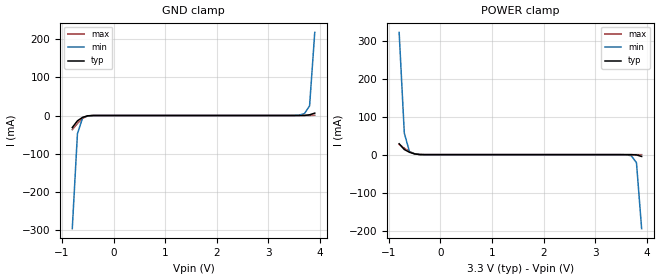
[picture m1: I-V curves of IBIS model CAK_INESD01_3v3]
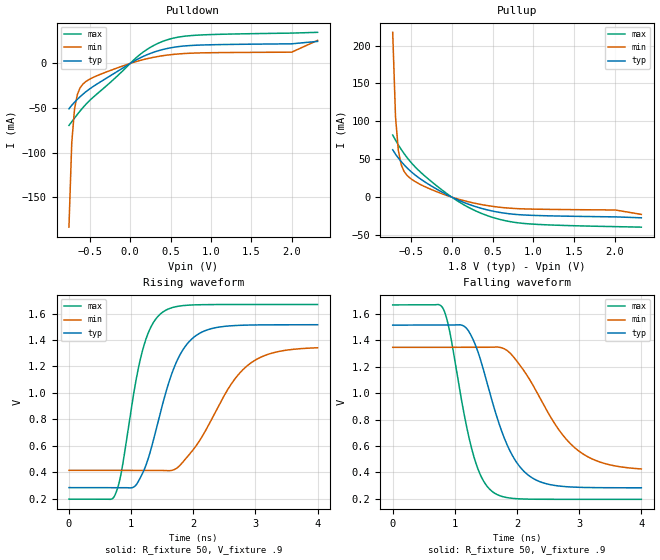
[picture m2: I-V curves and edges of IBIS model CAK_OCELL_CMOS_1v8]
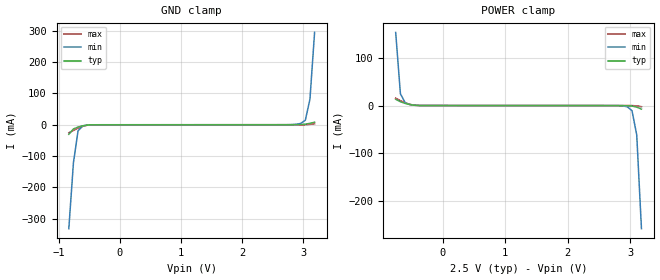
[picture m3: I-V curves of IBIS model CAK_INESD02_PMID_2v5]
|   This file is an IBIS representation of the   |
|   Integrated Device Technology Inc   |
|   IDT8T49N285I   |
|   FEMTOCLOCK NG OCTAL UNIVERSAL FREQUENCY TRANSLATOR   |
[IBIS Ver]   4.1
[File name]   8t49n285i.ibs
[File Rev]   1.0
[Date]   04 Dec 2014
[Source]   Originated at Integrated Device Technology, Inc.
[Disclaimer]
IDT hereby grants the user of this IBIS model a non-exclusive,
nontransferable license to use this IBIS model under the following terms.
Before using this IBIS model, the user should read this license.
If the user does not accept these terms,  the IBIS model should be
returned to IDT within 30 days.
   The user is granted this license only to use the IBIS model and
is not granted rights to sell, load, rent, lease or license the IBIS
model in whole or in part, or in modified form to anyone other than
user. User may modify the IBIS model to suit its specific
applications but rights to derivative works and such modifications
shall belong to IDT.
   This IBIS model is provided on an "AS IS" basis and IDT makes
absolutely no warranty with respect to the information contained
herein. IDT DISCLAIMS AND CUSTOMER WAIVES ALL WARRANTIES, EXPRESS
OR IMPLIED, INCLUDING WARRANTIES OF MERCHANTABILITY OR FITNESS FOR
A PARTICULAR PURPOSE. The entire risk as to quality and performance
is with the Customer. ACCORDINGLY, IN NO EVENT SHALL THE COMPANY BE
LIABLE FOR ANY DAMAGES, WHETHER IN CONTRACT OR TORT,INCLUDING ANY
LOST PROFITS OR OTHER INCIDENTAL, CONSEQUENTIAL, EXEMPLARY, OR
PUNITIVE DAMAGES ARISING OUT OF THE USE OR APPLICATION OF THE IBIS
model provided in this package. Further, IDT reserves the right to
make changes without notice to any product herein to improve
reliability, function, or design. IDT does not convey any license
under patent rights or any other intellectual property rights,
including those of third parties.
   IDT is not obligated to provide maintenance or support
for the licensed IBIS model.
[Copyright] Copyright 2014 by Integrated Device Technology, Inc.
[Component]   IDT8T49N285NLI
[Manufacturer] Integrated Device Technology, Inc.
[Package]
|LD QFN 56
|lead + wire   typ   min   max
R_pkg   294.15m   250.8m   337.5m
L_pkg   1.827nH   1.475nH   2.179nH
C_pkg   0.464pF   0.409pF   0.518pF
[Pin] signal_name model_name   R_pin   L_pin   C_pin
1  VCCA   POWER   337.50m   2.179n   0.518p
2  VCCA   POWER   323.05m   2.062n   0.500p
3  OSCI   CAK_INESD01   308.60m   1.944n   0.482p
4  OSCO   NC   294.15m   1.827n   0.464p
5  S_A0   CAK_INESD02_PD   279.70m   1.709n   0.446p
6  VEE   GND   265.25m   1.592n   0.427p
7  CLK0   CAK_INESD02_PD   250.80m   1.475n   0.409p
8  nCLKO   CAK_INESD02_PMID   250.80m   1.475n   0.409p
9  CLK1   CAK_INESD02_PD   265.25m   1.592n   0.427p
10 nCLK1   CAK_INESD02_PMID   279.70m   1.709n   0.446p
11 VCC   POWER   294.15m   1.827n   0.464p
12 SDATA   CAK_IOCMOS35OHM0   308.60m   1.944n   0.482p
13 SCLK   CAK_IOCMOS35OHM0   323.05m   2.062n   0.500p
14 VCCA   POWER   337.50m   2.179n   0.518p
15 VCCA   POWER   337.50m   2.179n   0.518p
16 VCCA   POWER   323.05m   2.062n   0.500p
17 VCC   POWER   308.60m   1.944n   0.482p
18 CAP1   NC   294.15m   1.827n   0.464p
19 CAP1_REF   NC   279.70m   1.709n   0.446p
20 VCCA   POWER   265.25m   1.592n   0.427p
21 GPI01   CAK_IOCMOS25OHM0   250.80m   1.475n   0.409p
22 VCCO3   POWER   250.80m   1.475n   0.409p
23 Q3   CAK_OCELL_MULTOUT   265.25m   1.592n   0.427p
24 nQ3   CAK_OCELL_MULTOUT   279.70m   1.709n   0.446p
25 GPIO0   CAK_IOCMOS25OHM0   294.15m   1.827n   0.464p
26 VCCO2   POWER   308.60m   1.944n   0.482p
27 Q2   CAK_OCELL_MULTOUT   323.05m   2.062n   0.500p
28 nQ2   CAK_OCELL_MULTOUT   337.50m   2.179n   0.518p
29 GPIO3   CAK_IOCMOS25OHM0   337.50m   2.179n   0.518p
30 nQ7   CAK_OCELL_MULTOUT   323.05m   2.062n   0.500p
31 Q7   CAK_OCELL_MULTOUT   308.60m   1.944n   0.482p
32 VCCO7   POWER   294.15m   1.827n   0.464p
33 nQ6   CAK_OCELL_MULTOUT   279.70m   1.709n   0.446p
34 Q6   CAK_OCELL_MULTOUT   265.25m   1.592n   0.427p
35 VCCO6   POWER   250.80m   1.475n   0.409p
36 nQ5   CAK_OCELL_MULTOUT   250.80m   1.475n   0.409p
37 Q5   CAK_OCELL_MULTOUT   265.25m   1.592n   0.427p
38 VCCO5   POWER   279.70m   1.709n   0.446p
39 nQ4   CAK_OCELL_MULTOUT   294.15m   1.827n   0.464p
40 Q4   CAK_OCELL_MULTOUT   308.60m   1.944n   0.482p
41 VCCO4   POWER   323.05m   2.062n   0.500p
42 GPIO2   CAK_IOCMOS25OHM0   337.50m   2.179n   0.518p
43 nQ1   CAK_OCELL_MULTOUT   337.50m   2.179n   0.518p
44 Q1   CAK_OCELL_MULTOUT   323.05m   2.062n   0.500p
45 VCCO1   POWER   308.60m   1.944n   0.482p
46 nRST   CAK_INESD01_PU_5   294.15m   1.827n   0.464p
47 nQ0   CAK_OCELL_MULTOUT   279.70m   1.709n   0.446p
48 Q0   CAK_OCELL_MULTOUT   265.25m   1.592n   0.427p
49 VCCO0   POWER   250.80m   1.475n   0.409p
50 nINT   OUTPUT_OD01   250.80m   1.475n   0.409p
51 VCCA   POWER   265.25m   1.592n   0.427p
52 CAP0_REF   NC   279.70m   1.709n   0.446p
53 CAP0   NC   294.15m   1.827n   0.464p
54 PLL_BYP   CAK_INESD01_PD_5   308.60m   1.944n   0.482p
55 VCCA   POWER   323.05m   2.062n   0.500p
56 VCCA   POWER   337.50m   2.179n   0.518p
[Diff Pin]   inv_pin vdiff   tdelay_typ   tdelay_min   tdelay_max
| Inputs
7   8   150mV   NA   NA   NA
9   10   150mV   NA   NA   NA
|Outputs
23   24   NA   0   0   0
27   28   NA   0   0   0
31   30   NA   0   0   0
34   33   NA   0   0   0
37   36   NA   0   0   0
40   39   NA   0   0   0
44   43   NA   0   0   0
48   47   NA   0   0   0
[Model Selector] CAK_INESD01
CAK_INESD01_2v5   Buffer selection for 2v5
CAK_INESD01_3v3   Buffer selection for 3v3
[Model Selector] CAK_INESD02_PD
CAK_INESD02_PD_2v5  Buffer selection for 2v5
CAK_INESD02_PD_3v3  Buffer selection for 3v3
[Model Selector] CAK_INESD02_PMID
CAK_INESD02_PMID_2v5  Buffer selection for 2v5
CAK_INESD02_PMID_3v3  Buffer selection for 3v3
[Model Selector] CAK_IOCMOS35OHM0
CAK_IOCMOS35OHM0_2v5  Buffer selection for 2v5
CAK_IOCMOS35OHM0_3v3  Buffer selection for 3v3
[Model Selector] CAK_IOCMOS25OHM0
CAK_IOCMOS25OHM0_2v5  Buffer selection for 2v5
CAK_IOCMOS25OHM0_3v3  Buffer selection for 3v3
[Model Selector] CAK_OCELL_MULTOUT
CAK_OCELL_LVPECL_2v5  Buffer selection for LVPECL 2.5V
CAK_OCELL_LVPECL_3v3  Buffer selection for LVPECL 3.3V
CAK_OCELL_LVDS_2v5   Buffer selection for LVDS 2.5V
CAK_OCELL_LVDS_3v3   Buffer selection for LVDS 3.3V
CAK_OCELL_CMOS_1v8   Buffer selection for CMOS 1.8V
CAK_OCELL_CMOS_2v5   Buffer selection for CMOS 2.5V
CAK_OCELL_CMOS_3v3   Buffer selection for CMOS 3.3V
CAK_OCELL_HCSL_2v5   Buffer selection for HCSL 2.5V
CAK_OCELL_HCSL_3v3   Buffer selection for HCSL 3.3V
[Model Selector] CAK_INESD01_PU_5
CAK_INESD01_PU_5_2v5  Buffer selection for 2v5
CAK_INESD01_PU_5_3v3  Buffer selection for 3v3
[Model Selector] OUTPUT_OD01
OUTPUT_OD01_2v5  Buffer selection for 2v5
OUTPUT_OD01_3v3  Buffer selection for 3v3
[Model Selector] CAK_INESD01_PD_5
CAK_INESD01_PD_5_2v5  Buffer selection for 2v5
CAK_INESD01_PD_5_3v3  Buffer selection for 3v3
| Models and submodels in the file (25): CAK_INESD01_3v3 (Input), CAK_INESD01_2v5 (Input), CAK_OCELL_CMOS_1v8 (Output), CAK_INESD02_PD_2v5 (Input), CAK_INESD02_PMID_2v5 (Input), CAK_IOCMOS35OHM0_2v5 (I/O), CAK_IOCMOS25OHM0_2v5 (I/O), CAK_OCELL_LVPECL_2v5 (Output_ECL), CAK_OCELL_CMOS_2v5 (Output), CAK_OCELL_LVDS_2v5 (Output), CAK_INESD01_PU_5_2v5 (Input), OUTPUT_OD01_2v5 (Open_drain), CAK_INESD01_PD_5_2v5 (Input), CAK_INESD02_PD_3v3 (Input), CAK_INESD02_PMID_3v3 (Input), CAK_IOCMOS35OHM0_3v3 (Output), CAK_IOCMOS25OHM0_3v3 (I/O), CAK_OCELL_LVPECL_3v3 (Output_ECL), CAK_OCELL_CMOS_3v3 (Output), CAK_OCELL_LVDS_3v3 (Output), CAK_INESD01_PU_5_3v3 (Input), OUTPUT_OD01_3v3 (Open_drain), CAK_INESD01_PD_5_3v3 (Input), CAK_OCELL_HCSL_3v3 (Open_source), CAK_OCELL_HCSL_2v5 (Open_source)
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[Model]   CAK_INESD01_3v3
Model_type   Input
Polarity   Non-Inverting
Vinl = 0.8V
Vinh = 2.0V
|   typ   min   max
C_comp   2pF   1.5pF   2.5pF
|   typ   min   max
[Voltage range]   3.3V   3.135V   3.465V
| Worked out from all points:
|   GND clamp passes 1 mA (typ) near -0.51 V on its own axis
|   POWER clamp passes 1 mA (typ) near -0.45 V on its own axis
[GND_clamp]
|Voltage   I (typ)   I (min)   I (max)
|Note, modeling breaks down at 250mA and above.  This is well beyond the functional   |
|operating range of the device.  Should this scenario occur, catastrophic failure and   |
|possible damage to the device and/or board is of higher concern than the I-V curve   |
|behavior.  The IBIS checker will flag currents in excess of 10A with warnings.  Lines   |
|with currents in excess of 0.35 A have been commented out.  The points still remain|
|available to the user if the user desires to use them.   |
|-3.30000e+00   -9.36876e+00   -7.41789e+00   -1.15553e+01
|-3.20000e+00   -8.98667e+00   -7.13115e+00   -1.10681e+01
|-3.10000e+00   -8.60459e+00   -6.84449e+00   -1.05809e+01
|-3.00000e+00   -8.22253e+00   -6.55791e+00   -1.00936e+01
|-2.90000e+00   -7.84049e+00   -6.27142e+00   -9.60637e+00
|-2.80000e+00   -7.45848e+00   -5.98504e+00   -9.11911e+00
|-2.70000e+00   -7.07651e+00   -5.69875e+00   -8.63183e+00
|-2.60000e+00   -6.69459e+00   -5.41259e+00   -8.14455e+00
|-2.50000e+00   -6.31272e+00   -5.12654e+00   -7.65728e+00
|-2.40000e+00   -5.93093e+00   -4.84063e+00   -7.17002e+00
|-2.30000e+00   -5.54921e+00   -4.55486e+00   -6.68278e+00
|-2.20000e+00   -5.16760e+00   -4.26925e+00   -6.19558e+00
|-2.10000e+00   -4.78610e+00   -3.98381e+00   -5.70844e+00
|-2.00000e+00   -4.40474e+00   -3.69855e+00   -5.22138e+00
|-1.90000e+00   -4.02353e+00   -3.41349e+00   -4.73442e+00
|-1.80000e+00   -3.64251e+00   -3.12864e+00   -4.24759e+00
|-1.70000e+00   -3.26171e+00   -2.84402e+00   -3.76091e+00
|-1.60000e+00   -2.88116e+00   -2.55965e+00   -3.27441e+00
|-1.50000e+00   -2.50090e+00   -2.27553e+00   -2.78813e+00
|-1.40000e+00   -2.12097e+00   -1.99169e+00   -2.30210e+00
|-1.30000e+00   -1.74142e+00   -1.70814e+00   -1.81640e+00
|-1.20000e+00   -1.36229e+00   -1.42490e+00   -1.33109e+00
|-1.10000e+00   -9.83643e-01   -1.14199e+00   -8.46264e-01
|-1.00000e+00   -6.05524e-01   -8.59476e-01   -3.62007e-01
|-9.00000e-01   -2.28002e-01   -5.77494e-01   -5.70861e-02
-800mV    -31.5mA    -296.3mA   -37.03mA
-700mV    -13.94mA   -47.89mA   -20.77mA
-600mV    -4.814mA   -5.925mA   -7.477mA
-500mV    -769.5uA   -876.2uA   -1.11mA
-400mV    -50.39uA   -91.12uA   -52.98uA
3.4V      929.4pA    7.738uA    18.23pA
3.6V      7.536uA    1.177mA    576.1pA
3.7V      200.6uA    4.949mA    206.1nA
3.8V      1.845mA    25.21mA    18.18uA
3.9V      6.193mA    217.6mA    563.4uA
| 4.00000e+00   1.34293e-02   5.06540e-01   3.84286e-03
| 4.10000e+00   2.85679e-02   7.94900e-01   1.06020e-02
| 4.20000e+00   2.42102e-01   1.08355e+00   2.05441e-02
| 4.30000e+00   6.27135e-01   1.37257e+00   3.02103e-02
| 4.40000e+00   1.01263e+00   1.66196e+00   7.70913e-02
| 4.50000e+00   1.39863e+00   1.95172e+00   5.37431e-01
| 4.60000e+00   1.78513e+00   2.24185e+00   1.03062e+00
| 4.70000e+00   2.17212e+00   2.53235e+00   1.52443e+00
| 4.80000e+00   2.55958e+00   2.82322e+00   2.01885e+00
| 4.90000e+00   2.94751e+00   3.11446e+00   2.51386e+00
| 5.00000e+00   3.33588e+00   3.40606e+00   3.00943e+00
| 5.10000e+00   3.72470e+00   3.69803e+00   3.50553e+00
| 5.20000e+00   4.11396e+00   3.99038e+00   4.00216e+00
| 5.30000e+00   4.50363e+00   4.28310e+00   4.49928e+00
| 5.40000e+00   4.89373e+00   4.57620e+00   4.99688e+00
| 5.50000e+00   5.28425e+00   4.86969e+00   5.49495e+00
| 5.60000e+00   5.67518e+00   5.16358e+00   5.99346e+00
| 5.70000e+00   6.06653e+00   5.45787e+00   6.49241e+00
| 5.80000e+00   6.45829e+00   5.75259e+00   6.99179e+00
| 5.90000e+00   6.85048e+00   6.04774e+00   7.49160e+00
| 6.00000e+00   7.24309e+00   6.34335e+00   7.99183e+00
| 6.10000e+00   7.63615e+00   6.63943e+00   8.49248e+00
| 6.20000e+00   8.02966e+00   6.93599e+00   8.99355e+00
| 6.30000e+00   8.42363e+00   7.23307e+00   9.49506e+00
| 6.40000e+00   8.81808e+00   7.53069e+00   9.99700e+00
| 6.50000e+00   9.21303e+00   7.82887e+00   1.04994e+01
| 6.60000e+00   9.60850e+00   8.12763e+00   1.10022e+01
[Power_clamp]
|Voltage   I (typ)   I (min)   I (max)
|Note, modeling breaks down at 250mA and above.  This is well beyond the functional   |
|operating range of the device.  Should this scenario occur, catastrophic failure and   |
|possible damage to the device and/or board is of higher concern than the I-V curve   |
|behavior.  The IBIS checker will flag currents in excess of 10A with warnings.  Lines   |
|with currents in excess of 0.35 A have been commented out.  The points still remain|
|available to the user if the user desires to use them.   |
|-3.30000e+00   9.60850e+00   7.63797e+00   1.18330e+01
|-3.20000e+00   9.21303e+00   7.34015e+00   1.13293e+01
|-3.10000e+00   8.81808e+00   7.04288e+00   1.08262e+01
|-3.00000e+00   8.42363e+00   6.74613e+00   1.03235e+01
|-2.90000e+00   8.02966e+00   6.44988e+00   9.82127e+00
|-2.80000e+00   7.63615e+00   6.15411e+00   9.31948e+00
|-2.70000e+00   7.24309e+00   5.85879e+00   8.81813e+00
|-2.60000e+00   6.85048e+00   5.56392e+00   8.31720e+00
|-2.50000e+00   6.45829e+00   5.26948e+00   7.81670e+00
|-2.40000e+00   6.06653e+00   4.97544e+00   7.31662e+00
|-2.30000e+00   5.67518e+00   4.68181e+00   6.81696e+00
|-2.20000e+00   5.28425e+00   4.38857e+00   6.31773e+00
|-2.10000e+00   4.89373e+00   4.09571e+00   5.81893e+00
|-2.00000e+00   4.50363e+00   3.80323e+00   5.32057e+00
|-1.90000e+00   4.11396e+00   3.51113e+00   4.82267e+00
|-1.80000e+00   3.72470e+00   3.21939e+00   4.32523e+00
|-1.70000e+00   3.33588e+00   2.92802e+00   3.82828e+00
|-1.60000e+00   2.94751e+00   2.63702e+00   3.33184e+00
|-1.50000e+00   2.55958e+00   2.34639e+00   2.83591e+00
|-1.40000e+00   2.17212e+00   2.05612e+00   2.34054e+00
|-1.30000e+00   1.78513e+00   1.76623e+00   1.84573e+00
|-1.20000e+00   1.39863e+00   1.47670e+00   1.35152e+00
|-1.10000e+00   1.01263e+00   1.18756e+00   8.57930e-01
|-1.00000e+00   6.27135e-01   8.98775e-01   3.64964e-01
|-9.00000e-01   2.42102e-01   6.10330e-01   4.20775e-02
-800mV    28.57mA    321.9mA    27.12mA
-700mV    13.43mA    56.36mA    16.78mA
-600mV    6.193mA    8.187mA    7.847mA
-500mV    1.845mA    2.071mA    2.293mA
-300mV    7.536uA    23.16uA    4.595uA
3.5V      -38.15nA   -37.11uA   -1.389nA
3.7V      -50.39uA   -3.041mA   -40.99nA
3.8V      -769.5uA   -21.19mA   -4.022uA
3.9V      -4.814mA   -194.9mA   -172.8uA
| 3.25758e+00   -2.17526e-02   -5.28437e-01   -1.11612e-02
| 3.33333e+00   -5.02557e-02   -7.41905e-01   -2.20995e-02
| 3.40909e+00   -2.62296e-01   -9.55738e-01   -3.45860e-02
| 3.48485e+00   -5.48283e-01   -1.16984e+00   -4.61839e-02
| 3.56061e+00   -8.34620e-01   -1.38416e+00   -9.03549e-02
| 3.63636e+00   -1.12128e+00   -1.59867e+00   -4.17005e-01
| 3.71212e+00   -1.40822e+00   -1.81336e+00   -7.83863e-01
| 3.78788e+00   -1.69544e+00   -2.02823e+00   -1.15106e+00
| 3.86364e+00   -1.98290e+00   -2.24326e+00   -1.51854e+00
| 3.93939e+00   -2.27059e+00   -2.45845e+00   -1.88629e+00
| 4.01515e+00   -2.55849e+00   -2.67380e+00   -2.25425e+00
| 4.09091e+00   -2.84658e+00   -2.88929e+00   -2.62240e+00
| 4.16667e+00   -3.13483e+00   -3.10491e+00   -2.99072e+00
| 4.24242e+00   -3.42324e+00   -3.32067e+00   -3.35917e+00
| 4.31818e+00   -3.71177e+00   -3.53656e+00   -3.72774e+00
| 4.39394e+00   -4.00043e+00   -3.75256e+00   -4.09641e+00
| 4.46970e+00   -4.28920e+00   -3.96868e+00   -4.46517e+00
| 4.54545e+00   -4.57807e+00   -4.18490e+00   -4.83401e+00
| 4.62121e+00   -4.86701e+00   -4.40122e+00   -5.20293e+00
| 4.69697e+00   -5.15604e+00   -4.61763e+00   -5.57191e+00
| 4.77273e+00   -5.44513e+00   -4.83413e+00   -5.94093e+00
| 4.84848e+00   -5.73428e+00   -5.05072e+00   -6.31000e+00
| 4.92424e+00   -6.02348e+00   -5.26738e+00   -6.67909e+00
| 5.00000e+00   -6.31272e+00   -5.48412e+00   -7.04821e+00
[Model]   CAK_OCELL_CMOS_1v8
Model_type   Output
Polarity   Non-Inverting
|   typ   min   max
C_comp   2pF   1.5pF   2.5pF
Vmeas = .9
Rref = 50
Cref = 0
Vref = .9
|   typ   min   max
[Voltage range]   1.8V   1.710V   1.890V
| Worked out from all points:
|   slope of the pulldown table from 0 to 0.27 V, typ, clamps not added: 22.7 ohm
|   slope of the pullup table from 0 to 0.27 V, typ, clamps not added: 22.9 ohm
|   rising waveform, R_fixture 50, V_fixture .9: 20-80 % time 472ps typ, 713ps min, 340ps max; typ from 0.284 V to 1.51 V
|   falling waveform, R_fixture 50, V_fixture .9: 20-80 % time 521ps typ, 753ps min, 370ps max; typ from 1.51 V to 0.284 V
[Pulldown]
|Voltage   I (typ)   I (min)   I (max)
|Note, modeling breaks down at 250mA and above.  This is well beyond the functional   |
|operating range of the device.  Should this scenario occur, catastrophic failure and   |
|possible damage to the device and/or board is of higher concern than the I-V curve   |
|behavior.  The IBIS checker will flag currents in excess of 10A with warnings.  Lines   |
|with currents in excess of 0.35 A have been commented out.  The points still remain|
|available to the user if the user desires to use them.   |
|-1.64000e+00   -8.45060e+00   -7.45572e+00   -9.66339e+00
|-1.48000e+00   -6.67178e+00   -6.12326e+00   -7.39014e+00
|-1.32000e+00   -4.89321e+00   -4.79099e+00   -5.11762e+00
|-1.16000e+00   -3.11502e+00   -3.45890e+00   -2.84539e+00
|-1.00000e+00   -1.33737e+00   -2.12700e+00   -5.73190e-01
|-9.99000e-01   -1.32626e+00   -2.11868e+00   -5.58990e-01
|-9.64529e-01   -9.43359e-01   -1.83177e+00   -1.98497e-01
|-9.30057e-01   -5.60487e-01   -1.54487e+00   -1.08372e-01
|-8.95586e-01   -2.31853e-01   -1.25801e+00   -8.77808e-02
|-8.61115e-01   -1.06256e-01   -9.71177e-01   -8.09581e-02
|-8.26644e-01   -6.89430e-02   -6.84381e-01   -7.68578e-02
|-7.92172e-01   -5.64352e-02   -4.00585e-01   -7.32011e-02
-757.7mV  -50.72mA   -183.3mA   -69.36mA
-723.2mV  -46.79mA   -89.01mA   -65.29mA
-688.8mV  -43.4mA    -50.99mA   -61.16mA
-654.3mV  -40.24mA   -34.84mA   -57.11mA
-619.8mV  -37.28mA   -27.27mA   -53.21mA
-550.9mV  -31.9mA    -20.42mA   -46.04mA
104.1mV   5.354mA    2.89mA     8.71mA
276.4mV   12.09mA    6.64mA     19.38mA
448.8mV   16.55mA    9.236mA    26.18mA
828mV     20.45mA    11.72mA    31.67mA
2.001V    21.99mA    12.65mA    33.99mA
2.321V    24.71mA    25.86mA    34.86mA
| 2.64060e+00   1.12686e-01   2.85444e+00   5.71416e-02
| 2.96040e+00   5.51975e+00   7.41138e+00   2.84717e+00
| 3.28020e+00   1.16082e+01   1.19723e+01   1.06308e+01
| 3.60000e+00   1.77021e+01   1.65374e+01   1.84207e+01
[Pullup]
|Voltage   I (typ)   I (min)   I (max)
|Note, modeling breaks down at 250mA and above.  This is well beyond the functional   |
|operating range of the device.  Should this scenario occur, catastrophic failure and   |
|possible damage to the device and/or board is of higher concern than the I-V curve   |
|behavior.  The IBIS checker will flag currents in excess of 10A with warnings.  Lines   |
|with currents in excess of 0.35 A have been commented out.  The points still remain|
|available to the user if the user desires to use them.   |
|-1.64000e+00   1.47162e+01   1.30180e+01   1.67914e+01
|-1.48000e+00   1.16627e+01   1.07308e+01   1.28878e+01
|-1.32000e+00   8.61028e+00   8.44452e+00   8.98520e+00
|-1.16000e+00   5.55874e+00   6.15894e+00   5.08347e+00
|-1.00000e+00   2.50796e+00   3.87398e+00   1.18251e+00
|-9.99000e-01   2.48890e+00   3.85970e+00   1.15813e+00
|-9.64529e-01   1.83169e+00   3.36748e+00   4.46554e-01
|-9.30057e-01   1.17449e+00   2.87526e+00   1.79719e-01
|-8.95586e-01   5.69042e-01   2.38303e+00   1.24495e-01
|-8.61115e-01   2.24186e-01   1.89075e+00   1.09758e-01
|-8.26644e-01   1.16045e-01   1.39834e+00   1.02419e-01
|-7.92172e-01   8.31335e-02   9.07732e-01   9.59623e-02
|-7.57701e-01   7.01040e-02   4.82756e-01   8.90038e-02
-723.2mV  62.45mA    217.4mA    81.87mA
-688.8mV  56.59mA    105.8mA    75.11mA
-654.3mV  51.54mA    61.61mA    68.83mA
-619.8mV  46.97mA    42.97mA    63.02mA
-585.3mV  42.79mA    34.1mA     57.63mA
-481.9mV  32.08mA    22.8mA     43.7mA
-240.6mV  14.08mA    9.573mA    19.72mA
69.61mV   -3.487mA   -2.304mA   -5.032mA
552.2mV   -19.55mA   -12.95mA   -28.42mA
1V        -24.13mA   -15.87mA   -35.71mA
2.001V    -26.07mA   -16.99mA   -38.95mA
2.321V    -27.3mA    -22.8mA    -39.65mA
| 2.64060e+00   -6.63615e-02   -1.53996e+00   -5.63223e-02
| 2.96040e+00   -3.10270e+00   -4.19870e+00   -1.55653e+00
| 3.28020e+00   -6.65517e+00   -6.85936e+00   -6.09630e+00
| 3.60000e+00   -1.02097e+01   -9.52145e+00   -1.06396e+01
[Ramp]
|   typ   min   max
dV/dt_r   0.74/0.473n   0.557/0.715n   0.883/0.339n
dV/dt_f   0.74/0.521n   0.553/0.755n   0.884/0.37n
R_load =   50.0000
[Rising Waveform]
R_fixture = 50
V_fixture = .9   |Vcc_typ
V_fixture_min = .855 |Vcc_min
V_fixture_max = .945 |Vcc_max
C_fixture = 0.0p
| Time   typ   min   max
0s        283.8mV    414.7mV    196.6mV
733.3ps   283.9mV    414.7mV    220.5mV
840ps     284mV      414.7mV    392.7mV
1.173ns   381.4mV    414.7mV    1.302V
1.316ns   567mV      414.9mV    1.496V
1.493ns   891.3mV    413.5mV    1.605V
1.773ns   1.277V     446.1mV    1.656V
2.12ns    1.455V     652.3mV    1.667V
2.893ns   1.513V     1.215V     1.668V
4ns       1.515V     1.341V     1.668V
[Falling Waveform]
R_fixture = 50
V_fixture = .9   |Vcc_typ
V_fixture_min = .855 |Vcc_min
V_fixture_max = .945 |Vcc_max
C_fixture = 0.0p
| Time   typ   min   max
0s        1.515V     1.347V     1.668V
813.3ps   1.515V     1.347V     1.639V
915.6ps   1.515V     1.347V     1.471V
1.28ns    1.419V     1.347V     563.3mV
1.431ns   1.225V     1.347V     361.5mV
1.604ns   932.5mV    1.349V     254.7mV
1.911ns   540.9mV    1.292V     204.7mV
2.262ns   353.9mV    1.056V     197.4mV
2.982ns   287.7mV    566.7mV    196.6mV
4ns       283.9mV    426.6mV    196.6mV
| 3.25758e+00   -1.32932e-02   -4.69388e-01   -6.85289e-03
| 3.33333e+00   -3.04767e-02   -6.80964e-01   -1.35047e-02
| 3.40909e+00   -1.97405e-01   -8.92761e-01   -2.10928e-02
| 3.48485e+00   -4.80463e-01   -1.10472e+00   -2.81524e-02
| 3.56061e+00   -7.63732e-01   -1.31681e+00   -5.47589e-02
| 3.63636e+00   -1.04719e+00   -1.52902e+00   -3.40294e-01
| 3.71212e+00   -1.33083e+00   -1.74134e+00   -7.02945e-01
| 3.78788e+00   -1.61464e+00   -1.95377e+00   -1.06580e+00
| 3.86364e+00   -1.89859e+00   -2.16629e+00   -1.42883e+00
| 3.93939e+00   -2.18269e+00   -2.37891e+00   -1.79201e+00
| 4.01515e+00   -2.46691e+00   -2.59162e+00   -2.15533e+00
| 4.09091e+00   -2.75125e+00   -2.80442e+00   -2.51876e+00
| 4.16667e+00   -3.03569e+00   -3.01730e+00   -2.88228e+00
| 4.24242e+00   -3.32022e+00   -3.23027e+00   -3.24589e+00
| 4.31818e+00   -3.60483e+00   -3.44330e+00   -3.60956e+00
| 4.39394e+00   -3.88952e+00   -3.65641e+00   -3.97330e+00
| 4.46970e+00   -4.17427e+00   -3.86959e+00   -4.33710e+00
| 4.54545e+00   -4.45909e+00   -4.08283e+00   -4.70095e+00
| 4.62121e+00   -4.74395e+00   -4.29613e+00   -5.06484e+00
| 4.69697e+00   -5.02886e+00   -4.50948e+00   -5.42878e+00
| 4.77273e+00   -5.31381e+00   -4.72289e+00   -5.79275e+00
| 4.84848e+00   -5.59879e+00   -4.93635e+00   -6.15675e+00
| 4.92424e+00   -5.88381e+00   -5.14986e+00   -6.52077e+00
| 5.00000e+00   -6.16885e+00   -5.36341e+00   -6.88480e+00
[Model] CAK_INESD02_PMID_2v5
Model_type   Input
Polarity   Non-Inverting
Vinl = 0.7V
Vinh = 1.7V
|   typ   min   max
C_comp   2pF   1.5pF   2.5pF
|   typ   min   max
[Voltage range]   2.5V   2.375V   2.625V
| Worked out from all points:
|   GND clamp passes 1 mA (typ) near -0.53 V on its own axis
|   POWER clamp passes 1 mA (typ) near -0.48 V on its own axis
[GND_clamp]
|Voltage   I (typ)   I (min)   I (max)
|Note, modeling breaks down at 250mA and above.  This is well beyond the functional   |
|operating range of the device.  Should this scenario occur, catastrophic failure and   |
|possible damage to the device and/or board is of higher concern than the I-V curve   |
|behavior.  The IBIS checker will flag currents in excess of 10A with warnings.  Lines   |
|with currents in excess of 0.35 A have been commented out.  The points still remain|
|available to the user if the user desires to use them.   |
|-2.50000e+00   -6.16895e+00   -5.01116e+00   -7.48559e+00
|-2.42424e+00   -5.88390e+00   -4.79768e+00   -7.12154e+00
|-2.34848e+00   -5.59889e+00   -4.58425e+00   -6.75750e+00
|-2.27273e+00   -5.31390e+00   -4.37088e+00   -6.39347e+00
|-2.19697e+00   -5.02895e+00   -4.15756e+00   -6.02946e+00
|-2.12121e+00   -4.74404e+00   -3.94430e+00   -5.66547e+00
|-2.04545e+00   -4.45918e+00   -3.73109e+00   -5.30151e+00
|-1.96970e+00   -4.17436e+00   -3.51796e+00   -4.93758e+00
|-1.89394e+00   -3.88961e+00   -3.30490e+00   -4.57370e+00
|-1.81818e+00   -3.60492e+00   -3.09191e+00   -4.20986e+00
|-1.74242e+00   -3.32030e+00   -2.87899e+00   -3.84609e+00
|-1.66667e+00   -3.03577e+00   -2.66616e+00   -3.48237e+00
|-1.59091e+00   -2.75133e+00   -2.45342e+00   -3.11872e+00
|-1.51515e+00   -2.46699e+00   -2.24077e+00   -2.75514e+00
|-1.43939e+00   -2.18277e+00   -2.02821e+00   -2.39164e+00
|-1.36364e+00   -1.89867e+00   -1.81575e+00   -2.02825e+00
|-1.28788e+00   -1.61471e+00   -1.60339e+00   -1.66497e+00
|-1.21212e+00   -1.33091e+00   -1.39114e+00   -1.30184e+00
|-1.13636e+00   -1.04727e+00   -1.17900e+00   -9.38864e-01
|-1.06061e+00   -7.63803e-01   -9.66990e-01   -5.76078e-01
|-9.84848e-01   -4.80532e-01   -7.55130e-01   -2.13501e-01
|-9.09091e-01   -1.97473e-01   -5.43466e-01   -3.76738e-02
-833.3mV  -30.54mA   -332.1mA   -25.65mA
-757.6mV  -13.36mA   -120.7mA   -18.55mA
-681.8mV  -7.383mA   -19.06mA   -11.06mA
-606.1mV  -3.294mA   -4.129mA   -5.066mA
-530.3mV  -997.9uA   -1.06mA    -1.479mA
-378.8mV  -81.26uA   -88.94uA   -93.18uA
2.727V    59.1uA     121uA      65.12uA
2.955V    596.4uA    4.136mA    85.43uA
3.03V     1.982mA    14.16mA    231.7uA
3.106V    4.438mA    81.6mA     1.173mA
3.182V    7.992mA    295.1mA    3.436mA
| 3.25758e+00   1.31680e-02   5.12428e-01   7.02139e-03
| 3.33333e+00   3.25724e-02   7.29725e-01   1.18654e-02
| 3.40909e+00   2.27266e-01   9.47135e-01   1.72034e-02
| 3.48485e+00   5.17409e-01   1.16468e+00   2.19847e-02
| 3.56061e+00   8.07728e-01   1.38237e+00   5.23158e-02
| 3.63636e+00   1.09824e+00   1.60020e+00   3.65997e-01
| 3.71212e+00   1.38894e+00   1.81817e+00   7.37335e-01
| 3.78788e+00   1.67983e+00   2.03629e+00   1.10891e+00
| 3.86364e+00   1.97091e+00   2.25454e+00   1.48073e+00
| 3.93939e+00   2.26217e+00   2.47294e+00   1.85278e+00
| 4.01515e+00   2.55361e+00   2.69148e+00   2.22506e+00
| 4.09091e+00   2.84523e+00   2.91016e+00   2.59755e+00
| 4.16667e+00   3.13703e+00   3.12898e+00   2.97026e+00
| 4.24242e+00   3.42899e+00   3.34794e+00   3.34317e+00
| 4.31818e+00   3.72112e+00   3.56704e+00   3.71628e+00
| 4.39394e+00   4.01342e+00   3.78629e+00   4.08959e+00
| 4.46970e+00   4.30588e+00   4.00567e+00   4.46308e+00
| 4.54545e+00   4.59850e+00   4.22520e+00   4.83676e+00
| 4.62121e+00   4.89128e+00   4.44488e+00   5.21061e+00
| 4.69697e+00   5.18421e+00   4.66471e+00   5.58464e+00
| 4.77273e+00   5.47731e+00   4.88468e+00   5.95883e+00
| 4.84848e+00   5.77057e+00   5.10481e+00   6.33320e+00
| 4.92424e+00   6.06399e+00   5.32510e+00   6.70773e+00
| 5.00000e+00   6.35756e+00   5.54554e+00   7.08242e+00
[Power_clamp]
|Voltage   I (typ)   I (min)   I (max)
|Note, modeling breaks down at 250mA and above.  This is well beyond the functional   |
|operating range of the device.  Should this scenario occur, catastrophic failure and   |
|possible damage to the device and/or board is of higher concern than the I-V curve   |
|behavior.  The IBIS checker will flag currents in excess of 10A with warnings.  Lines   |
|with currents in excess of 0.35 A have been commented out.  The points still remain|
|available to the user if the user desires to use them.   |
|-2.50000e+00   6.35756e+00   5.18189e+00   7.70102e+00
|-2.42424e+00   6.06399e+00   4.96171e+00   7.32606e+00
|-2.34848e+00   5.77057e+00   4.74168e+00   6.95126e+00
|-2.27273e+00   5.47731e+00   4.52180e+00   6.57663e+00
|-2.19697e+00   5.18421e+00   4.30207e+00   6.20215e+00
|-2.12121e+00   4.89128e+00   4.08249e+00   5.82785e+00
|-2.04545e+00   4.59850e+00   3.86306e+00   5.45371e+00
|-1.96970e+00   4.30588e+00   3.64376e+00   5.07974e+00
|-1.89394e+00   4.01342e+00   3.42461e+00   4.70595e+00
|-1.81818e+00   3.72112e+00   3.20560e+00   4.33234e+00
|-1.74242e+00   3.42899e+00   2.98673e+00   3.95891e+00
|-1.66667e+00   3.13703e+00   2.76800e+00   3.58567e+00
|-1.59091e+00   2.84523e+00   2.54941e+00   3.21263e+00
|-1.51515e+00   2.55361e+00   2.33097e+00   2.83979e+00
|-1.43939e+00   2.26217e+00   2.11266e+00   2.46715e+00
|-1.36364e+00   1.97091e+00   1.89450e+00   2.09473e+00
|-1.28788e+00   1.67983e+00   1.67647e+00   1.72254e+00
|-1.21212e+00   1.38894e+00   1.45859e+00   1.35057e+00
|-1.13636e+00   1.09824e+00   1.24086e+00   9.78833e-01
|-1.06061e+00   8.07728e-01   1.02326e+00   6.07339e-01
|-9.84848e-01   5.17409e-01   8.05803e-01   2.36085e-01
|-9.09091e-01   2.27266e-01   5.88473e-01   3.12941e-02
|-8.33333e-01   3.25724e-02   3.71194e-01   2.01370e-02
-757.6mV  13.17mA    153.4mA    15.42mA
-681.8mV  7.992mA    24.73mA    10.04mA
-606.1mV  4.438mA    6.043mA    5.618mA
-530.3mV  1.982mA    2.167mA    2.491mA
-303mV    67.49uA    68.92uA    77.83uA
2.727V    -58.92uA   -71.21uA   -65.12uA
2.955V    -222.7uA   -2.559mA   -77.6uA
3.03V     -997.9uA   -10.75mA   -119.7uA
3.106V    -3.295mA   -61.69mA   -506.7uA
3.182V    -7.383mA   -258.2mA   -2.426mA
